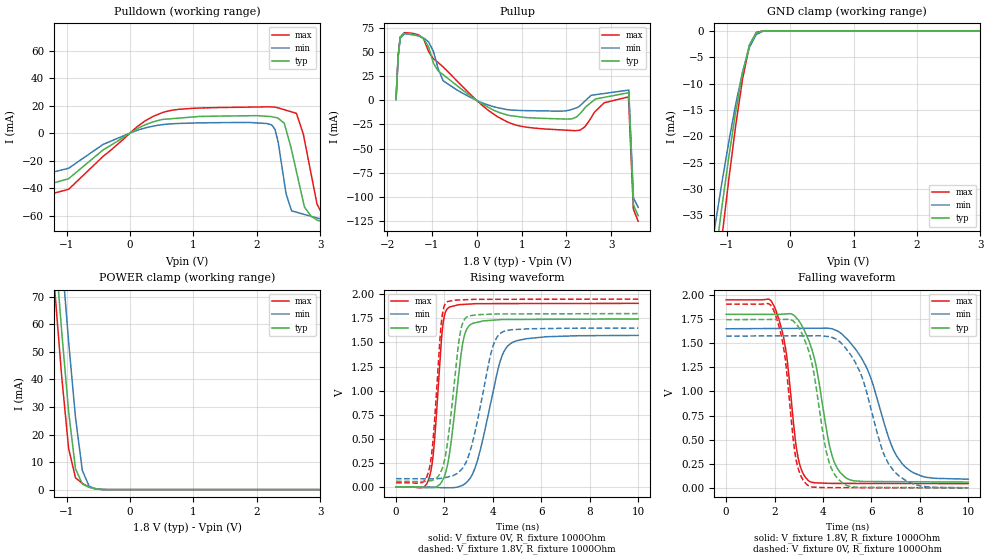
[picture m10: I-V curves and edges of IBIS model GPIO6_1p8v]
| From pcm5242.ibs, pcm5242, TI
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|   Model
[Model]   GPIO6_1p8v
Model_type   I/O
Polarity   Non-Inverting
Enable   Active-Low
Vinl = 0.54
Vinh = 1.26
Vmeas = 0.9
Vref = 0
Cref = 1pF
Rref = 1000000
|   typ   min   max
C_comp   1.487pF   1.458pF   1.501pF
[Voltage Range]   1.8   1.65   1.95
[Temperature Range]   27   105   -25
[Pullup Reference]   1.8   1.65   1.95
[Pulldown Reference]   -0   -0   -0
[Power Clamp Reference]   1.8   1.65   1.95
[GND Clamp Reference]   -0   -0   -0
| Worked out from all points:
|   slope of the pulldown table from 0 to 0.27 V, typ, clamps not added: 41.2 ohm
|   slope of the pullup table from 0 to 0.27 V, typ, clamps not added: 36.2 ohm
|   GND clamp passes 1 mA (typ) near -0.56 V on its own axis
|   POWER clamp passes 1 mA (typ) near -0.66 V on its own axis
|   falling waveform, V_fixture 1.8V, R_fixture 1000Ohm: 20-80 % time 777ps typ, 1.29ns min, 531ps max; typ from 1.8 V to 0.06 V
|   rising waveform, V_fixture 0V, R_fixture 1000Ohm: 20-80 % time 489ps typ, 845ps min, 323ps max; typ from 0 V to 1.74 V
|   rising waveform, V_fixture 1.8V, R_fixture 1000Ohm: 20-80 % time 470ps typ, 783ps min, 318ps max; typ from 0.06 V to 1.8 V
|   falling waveform, V_fixture 0V, R_fixture 1000Ohm: 20-80 % time 726ps typ, 1.16ns min, 509ps max; typ from 1.74 V to 0 V
[Pulldown]
|   Voltage   I(typ)   I(min)   I(max)
-1.8V     -18.87mA   -14.29mA   -22.86mA
-1.707V   -39.64mA   -31.51mA   -46.51mA
-1.506V   -40.12mA   -31.71mA   -47.41mA
-966.5mV  -33.16mA   -25.55mA   -40.87mA
518.8mV   9.953mA    6.174mA    15.01mA
2.3V      11.32mA    283.1uA    18.85mA
2.549V    -12.39mA   -56.54mA   15.42mA
2.752V    -53.77mA   -59.15mA   -4.979mA
2.95V     -63.16mA   -61.71mA   -51.68mA
3.383V    -67.48mA   -67.29mA   -67.92mA
3.492V    242.8mA    313.8mA    184.2mA
3.6V      283.7mA    359.8mA    218.7mA
[GND Clamp]
|   Voltage   I(typ)   I(min)   I(max)
-1.8V     -105.9mA   -88.79mA   -122.2mA
-1.182V   -43.15mA   -36.82mA   -50.61mA
-1.074V   -33.22mA   -28.66mA   -39.05mA
-966.5mV  -23.87mA   -20.97mA   -28.07mA
-858.5mV  -15.31mA   -13.91mA   -17.93mA
-750.5mV  -7.963mA   -7.777mA   -9.142mA
-642.5mV  -2.664mA   -3.129mA   -2.804mA
-534.5mV  -378.4uA   -687.8uA   -300.4uA
-426.5mV  -22.54uA   -76.81uA   -10.61uA
-318.5mV  -722.7nA   -5.54uA    -151.4nA
3.6V      0A         0A         0A
[Pullup]
|   Voltage   I(typ)   I(min)   I(max)
-1.8V     1.162mA    800.1uA    1.539mA
-1.754V   45.9mA     45.37mA    46.42mA
-1.707V   65.47mA    64.86mA    66.06mA
-1.614V   70.01mA    69.35mA    70.67mA
-1.074V   55.75mA    60.98mA    50.85mA
-750.5mV  26.86mA    20.54mA    34.94mA
880.1mV   -16.55mA   -10.23mA   -25.69mA
2.3V      -13.77mA   -5.516mA   -31.01mA
2.842V    3.234mA    7.277mA    -2.386mA
3.383V    8.074mA    10.78mA    3.709mA
3.492V    -106.2mA   -98.07mA   -113.1mA
3.6V      -119.9mA   -111.3mA   -125.8mA
[POWER Clamp]
|   Voltage   I(typ)   I(min)   I(max)
-1.8V     283.3mA    311.2mA    266.4mA
-1.182V   88.62mA    116.6mA    71.64mA
-1.074V   57.01mA    84.37mA    40.75mA
-966.5mV  28.23mA    53.67mA    14.9mA
-858.5mV  7.578mA    26.2mA     4.28mA
-750.5mV  2.019mA    6.936mA    2.253mA
-642.5mV  840.3uA    1.18mA     932.9uA
-534.5mV  214uA      297.3uA    193.5uA
-426.5mV  21.46uA    49.86uA    12.56uA
3.6V      0A         0A         0A
[Ramp]
R_load = 1000
|   typ   min   max
dV/dt_r   1.04652/4.88179e-10   0.944198/8.43878e-10   1.14357/3.22329e-10
dV/dt_f   1.04409/7.73999e-10   0.935932/1.28448e-09   1.14353/5.31087e-10
[Falling Waveform]
V_fixture = 1.8V
V_fixture_min = 1.65V
V_fixture_max = 1.95V
R_fixture = 1000Ohm
C_fixture = 0F
|   Time   V(typ)   V(min)   V(max)
0s        1.8V       1.65V      1.95V
1.975ns   1.8V       1.653V     1.887V
2.46ns    1.804V     1.654V     1.436V
2.979ns   1.741V     1.654V     300.9mV
3.392ns   1.539V     1.655V     75.87mV
4.372ns   333.4mV    1.65V      46.23mV
4.911ns   109.7mV    1.563V     46.03mV
5.809ns   66.08mV    1.242V     45.69mV
7.269ns   63.91mV    249.8mV    45.14mV
10ns      59.86mV    90.11mV    44.11mV
[Rising Waveform]
V_fixture = 0V
V_fixture_min = 0V
V_fixture_max = 0V
R_fixture = 1000Ohm
C_fixture = 0F
|   Time   V(typ)   V(min)   V(max)
0s        1.664nV    40.86nV    825.3pV
1.364ns   -6.664mV   640uV      92.9mV
1.575ns   -5.522mV   -2.435mV   446.6mV
1.93ns    74.87mV    -6.627mV   1.673V
2.162ns   279.8mV    -6.908mV   1.861V
2.724ns   1.447V     15.74mV    1.894V
3.048ns   1.681V     88.73mV    1.899V
4.299ns   1.737V     1.305V     1.904V
4.619ns   1.739V     1.466V     1.904V
10ns      1.744V     1.574V     1.906V
[Rising Waveform]
V_fixture = 1.8V
V_fixture_min = 1.65V
V_fixture_max = 1.95V
R_fixture = 1000Ohm
C_fixture = 0F
|   Time   V(typ)   V(min)   V(max)
0s        59.83mV    87.22mV    44.11mV
1.333ns   62.78mV    85.5mV     151.5mV
1.521ns   72.98mV    85.26mV    469.5mV
1.871ns   168.7mV    90.62mV    1.708V
2.084ns   391.4mV    101.5mV    1.918V
2.629ns   1.57V      165.4mV    1.942V
2.922ns   1.765V     276.4mV    1.944V
3.914ns   1.794V     1.383V     1.948V
4.299ns   1.796V     1.593V     1.948V
10ns      1.8V       1.65V      1.95V
[Falling Waveform]
|Gnd
V_fixture = 0V
V_fixture_min = 0V
V_fixture_max = 0V
R_fixture = 1000Ohm
C_fixture = 0F
|   Time   V(typ)   V(min)   V(max)
0s        1.744V     1.574V     1.906V
1.949ns   1.747V     1.576V     1.848V
2.408ns   1.748V     1.576V     1.396V
2.899ns   1.697V     1.577V     276.6mV
3.322ns   1.482V     1.577V     36.05mV
4.229ns   282.4mV    1.569V     2.679mV
4.809ns   48.87mV    1.486V     2.41mV
5.542ns   5.168mV    1.191V     2.07mV
6.908ns   3.592mV    180.1mV    1.436mV
10ns      19.81uV    1.454mV    1.496uV
